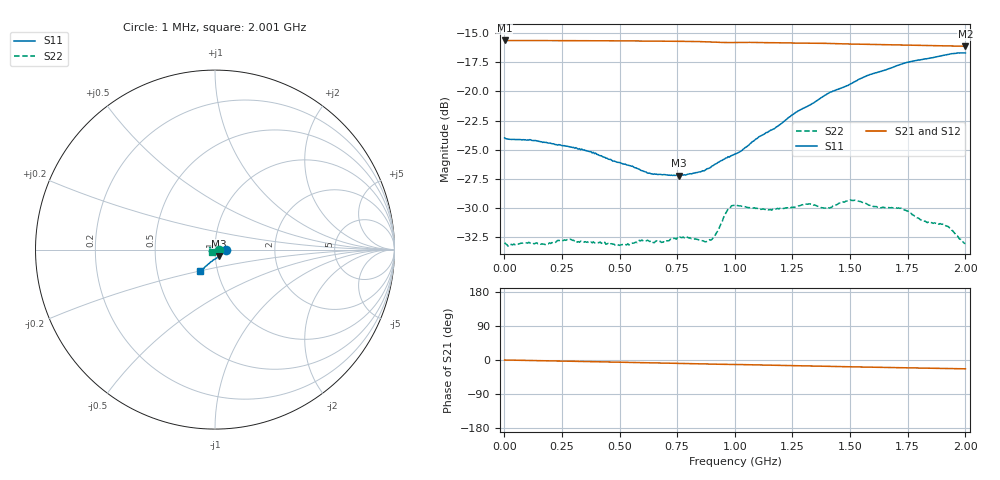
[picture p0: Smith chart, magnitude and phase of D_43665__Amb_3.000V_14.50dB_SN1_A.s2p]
! device id: 43665_
! dir: \\malibu\benchdata\1_engineers\tn_data\43665_75ohm\new\sparar\43665_\amb\3p000v\14p50db
! Serial: 1
! Insertion: A
! Temp: Amb
! VDD: 3.000V
! Attenuation Step: 14.50dB
! IDD: 1.452362e+00mA
! FILE NAME
! DATE 03-27-2009 08:36:55
! CORRECTED  DATA
#  Hz  S  RI  R  75
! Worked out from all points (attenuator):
!   401 points, 1 MHz to 2.001 GHz, reference 75 ohm
!   highest |S21| = -15.64 dB at 1 MHz (marker M1); lowest = -16.1 dB at 2.001 GHz (marker M2)
!   lowest |S11| = -27.2 dB at 756 MHz (marker M3), VSWR 1.09, Z = 78.4 - j5.78 ohm
!   |S11| at or under -10 dB: start of sweep to end of sweep
!   |S22| runs from -33.3 to -29.3 dB; largest |S21 - S12| = 0.00046
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1000000  0.0632 -0.000764  0.1652 -0.000218  0.1655 -0.000181  0.0225 -0.000197
1.81e8  0.0601 -0.00698  0.1649 -0.00593  0.1649 -0.00595  0.0194 0.0105
2.81e8  0.0568 -0.0119  0.1646 -0.00922  0.1647 -0.00924  0.0165 0.0163
3.36e8  0.0549 -0.0143  0.1644 -0.0111  0.1645 -0.0111  0.0135 0.0183
4.91e8  0.0449 -0.0214  0.1637 -0.0164  0.1638 -0.0164  0.00519 0.0213
5.91e8  0.0373 -0.0269  0.1629 -0.0198  0.163 -0.0197  -0.00172 0.0228
6.71e8  0.0305 -0.0319  0.1625 -0.0224  0.1625 -0.0223  -0.00589 0.0219
7.56e8  0.0234 -0.0368  0.1618 -0.0254  0.1619 -0.0253  -0.011 0.0207
8.91e8  0.00954 -0.0461  0.16 -0.0304  0.16 -0.0302  -0.0192 0.013
9.21e8  0.00614 -0.0487  0.1593 -0.0314  0.1594 -0.0312  -0.0222 0.0111
9.71e8  0.0015 -0.0525  0.1586 -0.0322  0.1587 -0.0321  -0.029 0.012
1.001e9  -0.00184 -0.0539  0.1585 -0.0329  0.1586 -0.0328  -0.0298 0.0128
1.151e9  -0.0177 -0.0653  0.157 -0.0381  0.1572 -0.0379  -0.0304 0.00683
1.336e9  -0.0372 -0.0805  0.1546 -0.044  0.1549 -0.0438  -0.0327 -0.00281
1.406e9  -0.0446 -0.0874  0.1535 -0.0465  0.1538 -0.0464  -0.0309 -0.00693
1.511e9  -0.0538 -0.0944  0.1516 -0.0493  0.1519 -0.0493  -0.0325 -0.0103
1.611e9  -0.0612 -0.1033  0.15 -0.0522  0.1503 -0.0524  -0.0296 -0.0124
1.671e9  -0.0662 -0.1063  0.1489 -0.0538  0.1491 -0.0538  -0.0292 -0.0127
1.721e9  -0.0698 -0.1105  0.148 -0.0551  0.1483 -0.0551  -0.0281 -0.0144
1.826e9  -0.0742 -0.1162  0.1463 -0.0576  0.1462 -0.0579  -0.0241 -0.0138
1.916e9  -0.0793 -0.1194  0.1448 -0.0597  0.1449 -0.0596  -0.0229 -0.0135
2.001e9  -0.0811 -0.1215  0.1434 -0.0615  0.1431 -0.0619  -0.019 -0.0117
